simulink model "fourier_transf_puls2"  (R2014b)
settings: Solver=ode45  StartTime=0.0  StopTime=10.0  RelTol=1e-3
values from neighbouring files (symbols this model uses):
  h = 1    [fourier_reihe_DFT_1.m]    (also in fourier_reihe_rechteck_1.m; fourier_reihe_rechteck_2.m; fourier_transf_puls_1.m; fourier_transf_puls_2.m = 2)
  N = 4*1024    (= 4096)    [ad_test_12.m]    (also in ad_test_2.m; ad_test_3.m; DA_wandler_spektr_1.m = 1000; DA_wandler_spektr_2.m = 1024)
  tau_abs = 25e-3    (= 0.025)    [fourier_transf_puls_1.m]    (also in fourier_transf_puls_2.m = 0.05)
  Ts = 1/fs    (= 0.00025)    [abtast_rate_1.m]    (also in ad_test_12.m = 0.0009765625; ad_test_2.m = 0.00048828125; ad_test_3.m = 0.00048828125; DA_wandler_spektr_1.m = 0.01)
  Tsig = N*Ts/nperioden    (= 0.0081466395112)    [ad_test_12.m]    (also in ad_test_2.m = 0.0093896713615; ad_test_3.m = 0.00937646507267; fourier_transf_puls_1.m = 0.32; fourier_transf_puls_2.m = 0.64)
undefined symbols (not defined in the file or in its folder): get
libraries: dspxfrm3 x1, simulink x1, dspsnks4 x1

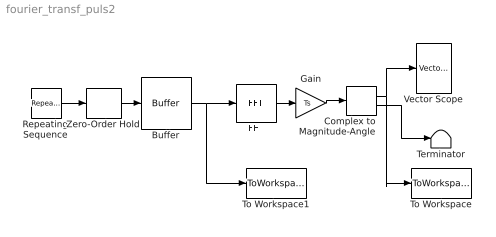
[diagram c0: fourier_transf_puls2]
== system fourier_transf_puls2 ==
  Buffer : Buffer  N=N  TreatMby1Signals=One channel
  Complex to Magnitude-Angle : ComplexToMagnitudeAngle
  FFT : dspxfrm3/FFT  CompMethod=Table lookup  TableOpt=NEW  TableOptActive=Speed  BitRevOrder=off  InheritFFTLength=on  FFTLength=64  WrapInput=on  RowConvenienceOn=on  FFTImplementation=Auto  SkipNorm=off  firstCoeffDataTypeStr=Inherit: Same word length as input  firstCoeffLastDataTypeStr=Inherit: Same word length as input  outputMin=[]  outputMax=[]  roundingMode=Floor  overflowMode=off
  Gain : Gain  Gain=Ts
  Repeating Sequence : simulink/Sources/Repeating Sequence  rep_seq_t=[0, tau_abs/2, tau_abs, Tsig ]  rep_seq_y=h*[0, 1, 0, 0]
  Terminator : Terminator
  To Workspace : ToWorkspace  VariableName=y  SaveFormat=Structure  SampleTime=-1
  To Workspace1 : ToWorkspace  VariableName=y1  SaveFormat=Structure  SampleTime=-1
  Vector Scope : dspsnks4/Vector Scope  ScopeProperties=on  Domain=Frequency  HorizSpan=1  DisplayProperties=off  AxisGrid=on  Memory=off  FrameNumber=on  AxisLegend=off  AxisZoom=off  OpenScopeAtSimStart=on  OpenScopeImmediately=off  FigPos=get(0,'defaultfigureposition')  AxisProperties=off  XUnits=Hertz  XRange=[0...Fs]  InheritXIncr=off  XIncr=1/1024  XLabel=Time  XLimit=User-defined  XMin=1.0667  XMax=1022.9333  XStart=0  YUnits=dB  YLabel=dB  LineProperties=off  XAxisParamsVer=6.9
  Zero-Order Hold : ZeroOrderHold  SampleTime=Ts
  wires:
  Repeating Sequence/1 -> Zero-Order Hold/1
  Zero-Order Hold/1 -> Buffer/1
  FFT/1 -> Gain/1
  Complex to Magnitude-Angle/1 -> To Workspace/1, Vector Scope/1
  Complex to Magnitude-Angle/2 -> Terminator/1
  Gain/1 -> Complex to Magnitude-Angle/1
  Buffer/1 -> To Workspace1/1, FFT/1
